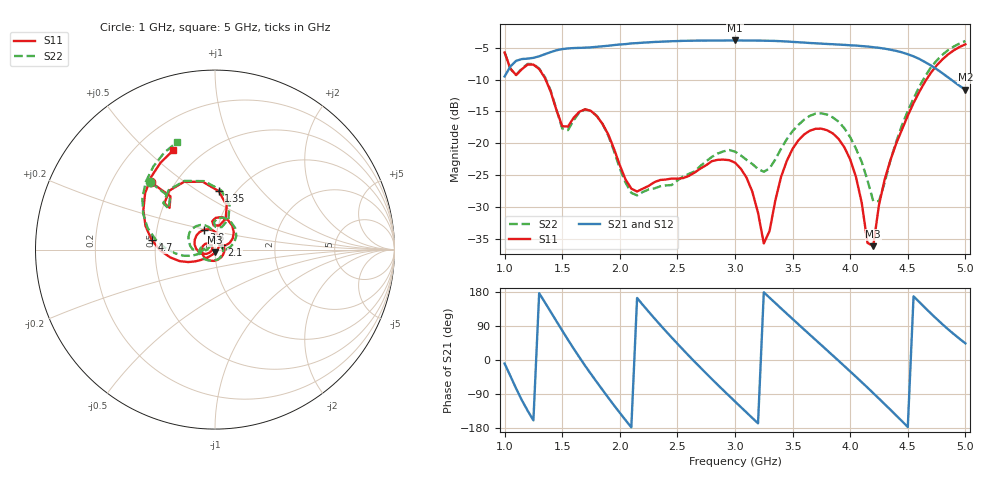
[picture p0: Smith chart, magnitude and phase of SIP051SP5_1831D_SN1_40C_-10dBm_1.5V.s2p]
# GHz  S  dB  R  50
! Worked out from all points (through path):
!   81 points, 1 GHz to 5 GHz, reference 50 ohm
!   highest |S21| = -3.84 dB at 3 GHz (marker M1); lowest = -11.6 dB at 5 GHz (marker M2)
!   lowest |S11| = -36.2 dB at 4.2 GHz (marker M3), VSWR 1.03, Z = 50.1 - j1.55 ohm
!   |S11| at or under -10 dB: 1.356 GHz to 4.661 GHz (3.305 GHz wide, 110 % of centre)
!   |S22| runs from -29.1 to -3.9 dB; largest |S21 - S12| = 0.0036
!   S11 on the Smith chart (normalised r, x): 1 GHz: 0.37, +0.38; 1.35 GHz: 0.84, +0.61; 2.1 GHz: 1.08, +0.05; 3.8 GHz: 0.86, +0.19; 4.7 GHz: 0.48, +0.06; 5 GHz: 0.35, +0.61
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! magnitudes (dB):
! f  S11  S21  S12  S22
! 1 GHz  -5.7  -9.5  -9.5  -5.7
! 1.1 GHz  -9.3  -7.0  -7.1  -9.3
! 1.35 GHz  -9.7  -6.0  -6.0  -9.6
! 1.5 GHz  -17.3  -5.2  -5.2  -17.7
! 1.7 GHz  -14.7  -5.0  -5.0  -14.7
! 1.85 GHz  -17.0  -4.7  -4.7  -17.0
! 2.1 GHz  -27.1  -4.3  -4.3  -27.8
! 2.35 GHz  -25.8  -4.0  -4.0  -26.8
! 3 GHz  -23.1  -3.8  -3.8  -21.3
! 3.15 GHz  -27.6  -3.8  -3.9  -23.3
! 3.25 GHz  -35.8  -3.9  -3.9  -24.5
! 3.45 GHz  -22.8  -4.0  -4.0  -19.3
! 3.7 GHz  -17.7  -4.3  -4.3  -15.3
! 3.8 GHz  -18.0  -4.4  -4.4  -15.5
! 4 GHz  -22.5  -4.6  -4.6  -19.1
! 4.1 GHz  -29.3  -4.7  -4.7  -22.9
! 4.15 GHz  -35.7  -4.8  -4.8  -25.8
! 4.2 GHz  -36.2  -4.9  -4.9  -29.1
! 4.25 GHz  -29.7  -5.0  -5.0  -29.1
! 4.35 GHz  -22.6  -5.3  -5.3  -22.6
! 4.7 GHz  -8.9  -7.8  -7.8  -8.1
! 5 GHz  -4.4  -11.6  -11.6  -3.9
